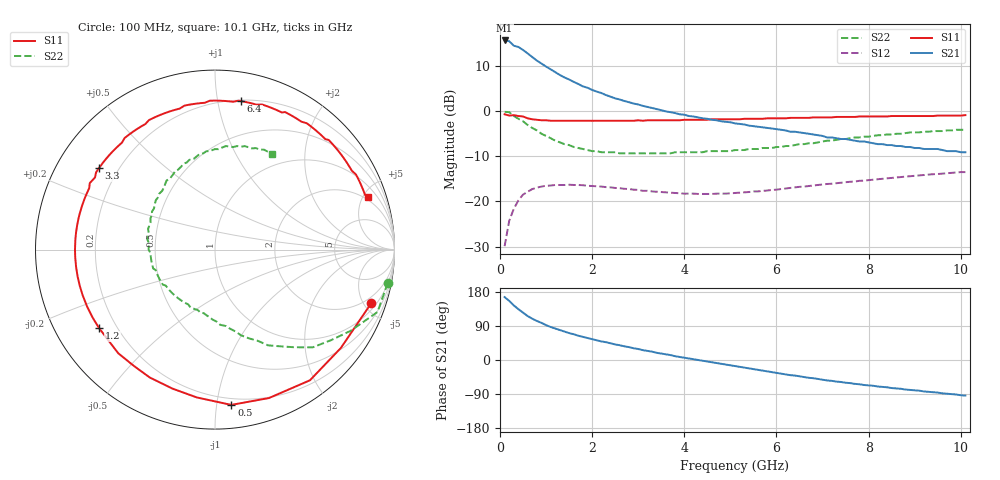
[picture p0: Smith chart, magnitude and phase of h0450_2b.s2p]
!HBFP-0450
!S and NOISE PARAMETERS at Vce=2V  Ic=2mA.  LAST UPDATED  09-04-98
# GHZ S MA R  50
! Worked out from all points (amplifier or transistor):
!   101 points, 100 MHz to 10.1 GHz, reference 50 ohm
!   highest |S21| = 15.6 dB at 100 MHz (marker M1)
!   |S21| within 3 dB of that: start of sweep to 615.9 MHz
!   unconditionally stable (mu >= 1): 3.31 GHz to end of sweep
!   at 1.7 GHz: K = 0.45, MSG = 11.2 dB, |S12| = -16.4 dB
!   at 5.1 GHz: K = 1.45, MAG = 3.7 dB, |S12| = -18.1 dB
!   at 10.1 GHz: K = 1.14, MAG = -0.1 dB, |S12| = -13.5 dB
!   lowest NFmin = 1.55 dB at 1.8 GHz
!   S11 on the Smith chart (normalised r, x): 100 MHz: 1.44, -5.62; 500 MHz: 0.15, -1.10; 1.2 GHz: 0.13, -0.30; 3.3 GHz: 0.13, +0.31; 6.4 GHz: 0.21, +1.17; 10.1 GHz: 1.76, +5.42
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0.1  0.92 -19.0  6.03 166.0  0.032 79.0  0.98 -11.0
0.2  0.89 -38.0  5.91 156.0  0.061 69.0  0.97 -21.0
0.3  0.9 -54.0  5.27 144.0  0.083 58.0  0.88 -31.0
0.4  0.88 -70.0  5.11 134.0  0.103 50.0  0.82 -38.0
0.5  0.87 -84.0  4.73 125.0  0.119 42.0  0.77 -45.0
0.6  0.83 -97.0  4.33 116.0  0.128 35.0  0.7 -51.0
0.7  0.81 -107.0  3.96 109.0  0.137 30.0  0.65 -56.0
0.8  0.8 -117.0  3.61 103.0  0.142 25.0  0.61 -61.0
1  0.79 -133.0  3.1 92.0  0.149 17.0  0.53 -69.0
1.2  0.78 -146.0  2.69 83.0  0.152 10.0  0.47 -76.0
1.5  0.78 -161.0  2.23 71.0  0.153 3.0  0.42 -86.0
1.8  0.78 -173.0  1.87 61.0  0.151 -3.0  0.38 -94.0
2.2  0.78 173.0  1.58 49.0  0.146 -9.0  0.35 -106.0
2.5  0.78 165.0  1.38 41.0  0.141 -12.0  0.35 -113.0
3.3  0.79 145.0  1.08 22.0  0.129 -18.0  0.34 -134.0
3.5  0.79 140.0  1.02 17.0  0.127 -19.0  0.34 -139.0
4.1  0.8 127.0  0.88 4.0  0.122 -20.0  0.35 -153.0
5.1  0.81 106.0  0.73 -16.0  0.124 -20.0  0.37 -180.0
6.4  0.84 80.0  0.59 -41.0  0.143 -24.0  0.42 143.0
6.8  0.85 72.0  0.55 -48.0  0.15 -27.0  0.44 132.0
8.5  0.88 44.0  0.42 -74.0  0.182 -43.0  0.55 93.0
10.1  0.9 19.0  0.35 -94.0  0.211 -64.0  0.62 59.0
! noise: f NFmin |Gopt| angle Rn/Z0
1.8  1.55  0.58  153  0.08
2  1.59  0.62  163  0.06
2.5  1.85  0.67  -178  0.05
3.5  2.23  0.74  -148  0.18
4  2.42  0.78  -135  0.37
5  2.89  0.8  -111  1.07
5.5  3.21  0.82  -100  1.66
7  3.56  0.87  -69  4.12
8  4.05  0.88  -52  6.31
10  4.68  0.88  -21  9.9
